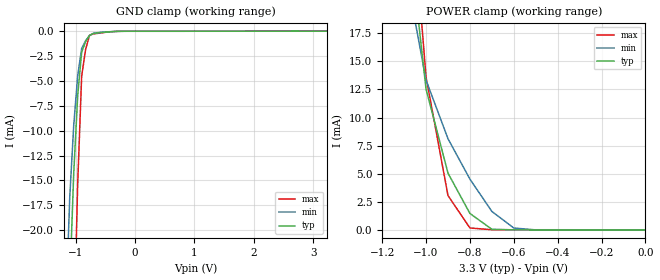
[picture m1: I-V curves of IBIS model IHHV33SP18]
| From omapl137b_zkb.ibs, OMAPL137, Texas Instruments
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|   Model Cell IHHV33SP18
|IHHV33SP18
[Model]   IHHV33SP18
Model_type   Input
Polarity   Non-Inverting
Vinl =  0.8V
Vinh =  2V
C_comp   0.7152039p   0.6019296p   0.8260735p
[Model Spec]
Vinl   0.8V   0.8V   0.8V
Vinh   2V   2V   2V
[Temperature Range]   25   125   -40
[Voltage Range]   3.3   2.97   3.63
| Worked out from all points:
|   GND clamp passes 1 mA (typ) near -0.83 V on its own axis
|   POWER clamp passes 1 mA (typ) near -0.77 V on its own axis
[POWER_clamp]
|   voltage   I(typ)   I(min)   I(max)
-3.3V     753mA      912.7mA    835.8mA
-1.067V   24.25mA    20.34mA    29.77mA
-1.033V   18.39mA    16.84mA    21.69mA
-1V       12.53mA    13.33mA    13.61mA
-900mV    5.059mA    8.121mA    3.065mA
-800mV    1.468mA    4.525mA    178.1uA
-700mV    65.34uA    1.651mA    22.6uA
-600mV    7.591uA    176.3uA    21.08uA
-500mV    6.792uA    7.103uA    20.51uA
-11.55fV  6.099uA    1.227uA    18.16uA
[GND_clamp]
|   voltage   I(typ)   I(min)   I(max)
-3.3V     -689.7mA   -840.2mA   -1.042A
-1.167V   -41.02mA   -28mA      -77.75mA
-1.1V     -25.47mA   -16.67mA   -52.12mA
-1.033V   -14.29mA   -9.465mA   -31.23mA
-966.7mV  -6.506mA   -4.488mA   -15.37mA
-900mV    -2.115mA   -1.737mA   -4.542mA
-833.3mV  -1.041mA   -948.6uA   -1.832mA
-766.7mV  -408.9uA   -436.9uA   -407.6uA
-700mV    -219.2uA   -201.9uA   -270.2uA
-233.3mV  -3.882uA   -5.236uA   -2.953uA
3.233V    6.019uA    1.284uA    16.64uA
